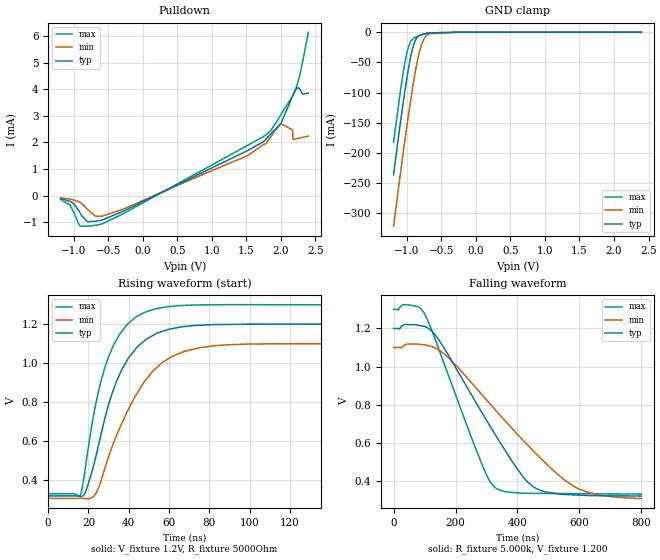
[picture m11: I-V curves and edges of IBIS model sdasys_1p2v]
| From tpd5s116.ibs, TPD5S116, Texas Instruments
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[Model]   sdasys_1p2v
Model_type   I/O_open_drain
Polarity   Non-Inverting
Enable   Active-Low
Vinl = .0902
Vinh = 0.91
Vmeas = 0.6
Vref = 1.2
Cref = 15pF
Rref = 5000
|   typ   min   max
|   (nom PVT)   (slow PVT)   (fast PVT)
C_comp   1.0804p   0.9332p   1.0809p
| Where nom  PVT is Nominal Process, 1.2V, 27C
|   Fast PVT is Strong Process,  1.3V, -40C
|   Slow PVT is Weak Process,   1.1V, 125C
[Voltage Range]   1.2   1.1   1.3
[Temperature Range]   27   125   -40
[Pullup Reference]   1.2   1.1   1.3
[Pulldown Reference]   -0   -0   -0
[Power Clamp Reference]   1.2   1.1   1.3
[GND Clamp Reference]   -0   -0   -0
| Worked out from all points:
|   slope of the pulldown table from 0 to 0.18 V, typ, clamps not added: 787 ohm
|   falling waveform, R_fixture 5.000k, V_fixture 1.200: 20-80 % time 196ns typ, 272ns min, 134ns max; typ from 1.2 V to 0.32 V
|   rising waveform, V_fixture 1.2V, R_fixture 5000Ohm: 20-80 % time 16.6ns typ, 22.3ns min, 13.9ns max; typ from 0.318 V to 1.2 V
[Pulldown]
|   Voltage   I(typ)   I(min)   I(max)
-1.193V   -116.5uA   -90.15uA   -144.3uA
-1.052V   -218.3uA   -137.4uA   -366.9uA
-922.8mV  -582.9uA   -244.9uA   -1.114mA
-804mV    -986.2uA   -517.8uA   -1.156mA
-591.6mV  -921.7uA   -777.8uA   -1.071mA
1.788V    2.128mA    1.964mA    2.292mA
1.997V    2.704mA    2.697mA    3.032mA
2.162V    3.703mA    2.475mA    3.721mA
2.177V    3.794mA    2.108mA    3.785mA
2.267V    4.03mA     2.16mA     4.468mA
2.314V    3.812mA    2.188mA    5.025mA
2.396V    3.854mA    2.233mA    6.14mA
[GND Clamp]
|   Voltage   I(typ)   I(min)   I(max)
-1.193V   -236.2mA   -321.7mA   -182.2mA
-1.081V   -139.5mA   -223.3mA   -87.96mA
-1.038V   -104.6mA   -186.7mA   -56.37mA
-991.2mV  -69.73mA   -148.3mA   -29.53mA
-937.2mV  -36.17mA   -106.5mA   -13.73mA
-879.6mV  -13.79mA   -66.41mA   -8.401mA
-829.2mV  -6.112mA   -37.58mA   -5.845mA
-793.2mV  -3.947mA   -22.16mA   -4.356mA
-746.4mV  -2.422mA   -9.645mA   -2.757mA
-714mV    -1.711mA   -5.18mA    -1.884mA
-300mV    -404.5nA   -3.869uA   -37.76nA
2.396V    0A         0A         0A
[Ramp]
R_load = 5000
|   typ   min   max
dV/dt_r   0.528844/1.66277e-08   0.476504/2.22673e-08   0.582092/1.38575e-08
dV/dt_f   0.528227/1.95525e-07   0.471298/2.71502e-07   0.582021/1.33276e-07
[Falling Waveform]
R_fixture = 5.000k
V_fixture = 1.200
V_fixture_min = 1.100
V_fixture_max = 1.300
C_fixture = 0.000
|  time   V(typ)   V(min)   V(max)
0s        1.2V       1.1V       1.3V
47.73ns   1.22V      1.118V     1.324V
97.1ns    1.212V     1.114V     1.285V
142.3ns   1.149V     1.091V     1.108V
286.2ns   755.3mV    850.8mV    483.3mV
329.5ns   638.6mV    770.6mV    362.4mV
419.1ns   418.7mV    611.1mV    334.1mV
477.5ns   347.4mV    514.1mV    333.5mV
622ns     323mV      342mV      331.9mV
800ns     319.6mV    305.8mV    330mV
[Rising Waveform]
V_fixture = 1.2V
V_fixture_min = 1.1V
V_fixture_max = 1.3V
R_fixture = 5000Ohm
C_fixture = 0F
|   Time   V(typ)   V(min)   V(max)
0s        318.4mV    305.8mV    329.8mV
15.8ns    316.3mV    305.9mV    320.2mV
18.29ns   333.6mV    305mV      450.1mV
23.45ns   511.4mV    326.8mV    780.9mV
27.82ns   702.4mV    448.9mV    966.5mV
32.45ns   864.9mV    590.1mV    1.093V
44.48ns   1.086V     850.9mV    1.242V
58.77ns   1.17V      1.017V     1.289V
104.3ns   1.2V       1.099V     1.3V
800ns     1.2V       1.1V       1.3V
